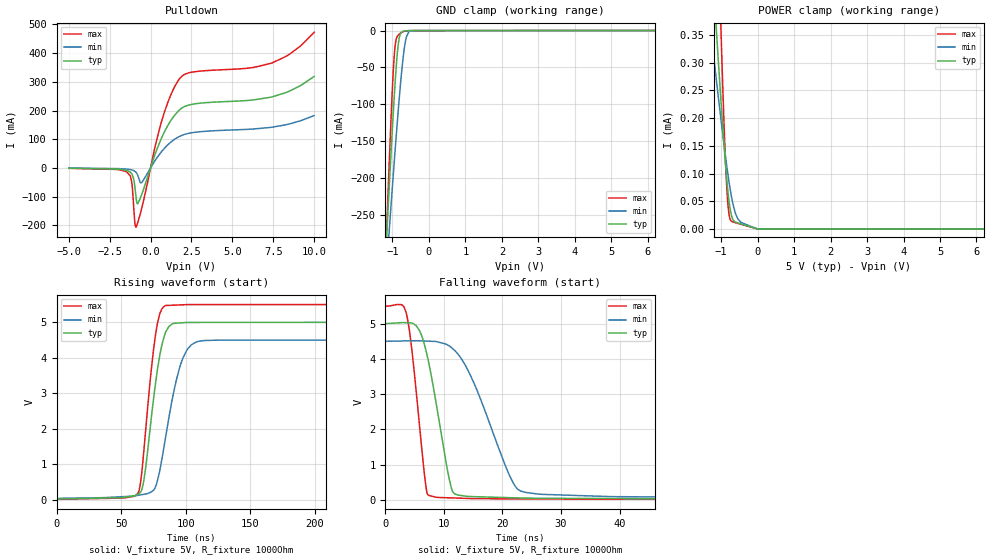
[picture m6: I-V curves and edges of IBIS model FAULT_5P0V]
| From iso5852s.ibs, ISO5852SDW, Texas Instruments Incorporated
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|   Model FAULT_5P0V
[Model]   FAULT_5P0V
Model_type   Open_drain
Polarity   Non-Inverting
Vmeas = 2.5
Vref = 5
Cref = 5pF
Rref = 1000
|   typ   min   max
|   (nom PVT)   (slow PVT)   (fast PVT)
C_comp   1.192p   1.159p   1.291p
|C_comp (ON state)   1.395p   1.317p   1.529p
|C_comp (OFF state)   1.192p   1.159p   1.291p
| Where   nom PVT is  Nominal Process, 5.0V, 27C
|   Fast PVT is Strong Process, 5.5V, -40C
|   Slow PVT is Weak Process, 4.5V, 150C
[Voltage Range]   5   4.5   5.5
[Temperature Range]   27   150   -40
[Pullup Reference]   5   4.5   5.5
[Pulldown Reference]   0   0   0
[Power Clamp Reference]   5   4.5   5.5
[GND Clamp Reference]   0   0   0
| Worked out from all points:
|   slope of the pulldown table from 0 to 0.75 V, typ, clamps not added: 6.57 ohm
|   GND clamp passes 1 mA (typ) near -0.71 V on its own axis
|   falling waveform, V_fixture 5V, R_fixture 1000Ohm: 20-80 % time 3.16ns typ, 6.26ns min, 2.01ns max; typ from 5 V to 0.028 V
|   rising waveform, V_fixture 5V, R_fixture 1000Ohm: 20-80 % time 10.3ns typ, 13.9ns min, 8.81ns max; typ from 0.028 V to 5 V
[Pulldown]
|   Voltage   I(typ)   I(min)   I(max)
-5V       -1.123mA   -755.9uA   -1.38mA
-1.475V   -8.517mA   -4.168mA   -12.99mA
-1.175V   -18.71mA   -6.76mA    -41.85mA
-1.115V   -24.24mA   -7.702mA   -67.88mA
-965mV    -63.8mA    -11.66mA   -188.6mA
-890mV    -101.9mA   -15.41mA   -206.5mA
-785mV    -125mA     -25.58mA   -191mA
-560mV    -95.32mA   -51.9mA    -144.7mA
685mV     106.1mA    57.68mA    164.6mA
1.765V    201.9mA    109.6mA    310.6mA
7.33V     246.2mA    141mA      364mA
10V       318.6mA    182.4mA    472.4mA
[GND Clamp]
|   Voltage   I(typ)   I(min)   I(max)
-5V       -4.292A    -3.18A     -5.824A
-1.16V    -279.2mA   -320mA     -270mA
-1.13V    -250.3mA   -299.1mA   -230.8mA
-1.085V   -207.7mA   -267.9mA   -173.5mA
-1.01V    -139.1mA   -216.7mA   -86.02mA
-950mV    -88.16mA   -176.7mA   -32.91mA
-905mV    -54.25mA   -147.4mA   -13.3mA
-830mV    -14.48mA   -100.9mA   -5.549mA
-710mV    -1.036mA   -37.32mA   -1.7mA
-620mV    -279uA     -8.956mA   -467.1uA
-410mV    -109.5uA   -166.9uA   -110.9uA
10V       0A         0A         0A
[POWER Clamp]
|   Voltage   I(typ)   I(min)   I(max)
-5V       185.6mA    66.98mA    302.3mA
-3.35V    2.813mA    1.63mA     6.063mA
-1.25V    483.8uA    338.2uA    914.2uA
-1.13V    357.7uA    268.3uA    636.2uA
-1.01V    236uA      200.4uA    369.5uA
-890mV    124.5uA    136uA      136.4uA
-830mV    77.82uA    106.1uA    58uA
-770mV    43.13uA    78.94uA    21.38uA
-680mV    17.22uA    46.14uA    12.69uA
-470mV    9.384uA    12.79uA    8.679uA
-5mV      77.67nA    104.1nA    72.22nA
10V       0A         0A         0A
[Ramp]
R_load = 1000
|   typ   min   max
dV/dt_r   2.98341/1.02367e-08   2.67222/1.38873e-08   3.28837/8.76833e-09
dV/dt_f   2.9834/3.15808e-09   2.67208/6.26205e-09   3.28837/2.00429e-09
[Falling Waveform]
V_fixture = 5V
V_fixture_min = 4.5V
V_fixture_max = 5.5V
R_fixture = 1000Ohm
C_fixture = 0F
|   Time   V(typ)   V(min)   V(max)
0s        5V         4.5V       5.5V
3.56ns    5.027V     4.511V     5.32V
4.599ns   5.014V     4.514V     4.189V
7.018ns   4.2V       4.507V     310.6mV
8.627ns   2.816V     4.496V     80.48mV
10.94ns   589.1mV    4.368V     62.07mV
11.84ns   175.7mV    4.246V     57.1mV
21.87ns   63.45mV    481.8mV    33.21mV
25.98ns   50.82mV    171.5mV    30.37mV
299.9ns   27.66mV    46.53mV    19.39mV
[Rising Waveform]
V_fixture = 5V
V_fixture_min = 4.5V
V_fixture_max = 5.5V
R_fixture = 1000Ohm
C_fixture = 0F
|   Time   V(typ)   V(min)   V(max)
0s        27.65mV    46.3mV     19.39mV
63.12ns   161.1mV    134.2mV    196.1mV
65.26ns   234mV      147.2mV    556.1mV
67.65ns   573.4mV    161.8mV    1.413V
76.52ns   3.258V     369.1mV    4.626V
79.62ns   4.005V     777.3mV    5.202V
83.79ns   4.647V     1.631V     5.458V
95.62ns   4.982V     3.765V     5.489V
108ns     4.996V     4.442V     5.498V
299.9ns   5V         4.5V       5.5V
